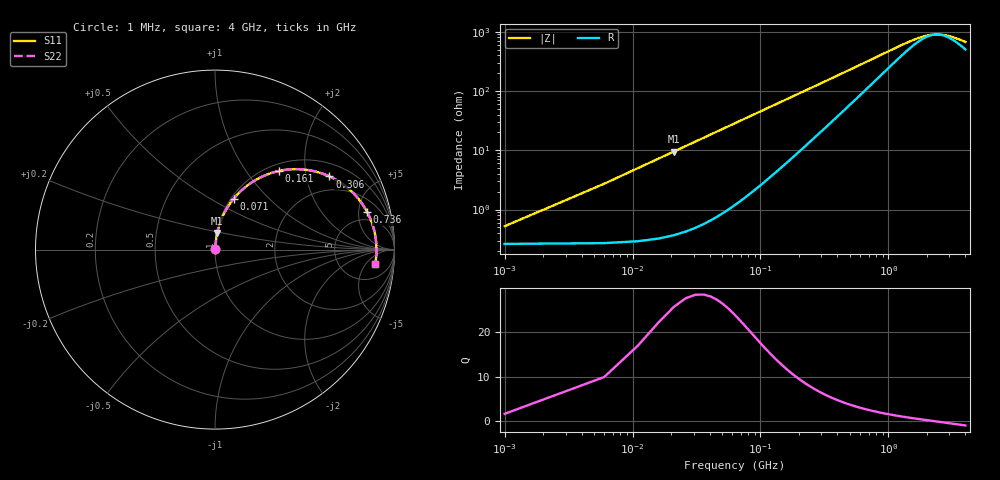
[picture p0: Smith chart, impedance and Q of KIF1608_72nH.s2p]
# MHz S RI R 50
!Freq ReS11 ImS11 ReS21 ImS21 ReS12 ImS12 ReS22 ImS22
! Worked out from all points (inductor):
!   801 points, 1 MHz to 4 GHz, reference 50 ohm
!   read as one part in series: L = 71.9 nH near 21 MHz
!   highest Q = 24.3 at 21 MHz (marker M1), where L = 71.9 nH
!   self-resonance near 2.396 GHz
!   S11 on the Smith chart (normalised r, x): 1 MHz: 1.01, +0.01; 71 MHz: 1.03, +0.64; 161 MHz: 1.12, +1.45; 306 MHz: 1.44, +2.74; 736 MHz: 3.58, +6.28; 4 GHz: 11, -9
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1  0.00265 0.0045  0.9974 -0.0045  0.9974 -0.0045  0.00265 0.0045
11  0.00536 0.0493  0.9946 -0.0493  0.9946 -0.0493  0.00536 0.0493
21  0.0125 0.0934  0.9875 -0.0934  0.9875 -0.0934  0.0125 0.0934
26  0.0177 0.1149  0.9823 -0.1149  0.9823 -0.1149  0.0177 0.1149
36  0.031 0.1567  0.969 -0.1567  0.969 -0.1567  0.031 0.1567
51  0.0578 0.2152  0.9422 -0.2152  0.9422 -0.2152  0.0578 0.2152
71  0.1036 0.2832  0.8964 -0.2832  0.8964 -0.2832  0.1036 0.2832
111  0.2151 0.3812  0.7849 -0.3812  0.7849 -0.3812  0.2151 0.3812
161  0.3579 0.4385  0.6421 -0.4385  0.6421 -0.4385  0.3579 0.4385
231  0.52 0.4431  0.48 -0.4431  0.48 -0.4431  0.52 0.4431
306  0.6377 0.4078  0.3623 -0.4078  0.3623 -0.4078  0.6377 0.4078
376  0.7098 0.3664  0.2902 -0.3664  0.2902 -0.3664  0.7098 0.3664
456  0.7639 0.3214  0.2361 -0.3214  0.2361 -0.3214  0.7639 0.3214
671  0.8369 0.2289  0.1631 -0.2289  0.1631 -0.2289  0.8369 0.2289
736  0.8486 0.2079  0.1514 -0.2079  0.1514 -0.2079  0.8486 0.2079
1021  0.8773 0.1401  0.1227 -0.1401  0.1227 -0.1401  0.8773 0.1401
1336  0.8903 0.0915  0.1097 -0.0915  0.1097 -0.0915  0.8903 0.0915
1666  0.8963 0.0553  0.1037 -0.0553  0.1037 -0.0553  0.8963 0.0553
2001  0.8989 0.0271  0.1011 -0.0271  0.1011 -0.0271  0.8989 0.0271
2671  0.8994 -0.0163  0.1006 0.0163  0.1006 0.0163  0.8994 -0.0163
3336  0.8969 -0.0503  0.1031 0.0503  0.1031 0.0503  0.8969 -0.0503
4000  0.8927 -0.0794  0.1073 0.0794  0.1073 0.0794  0.8927 -0.0794
